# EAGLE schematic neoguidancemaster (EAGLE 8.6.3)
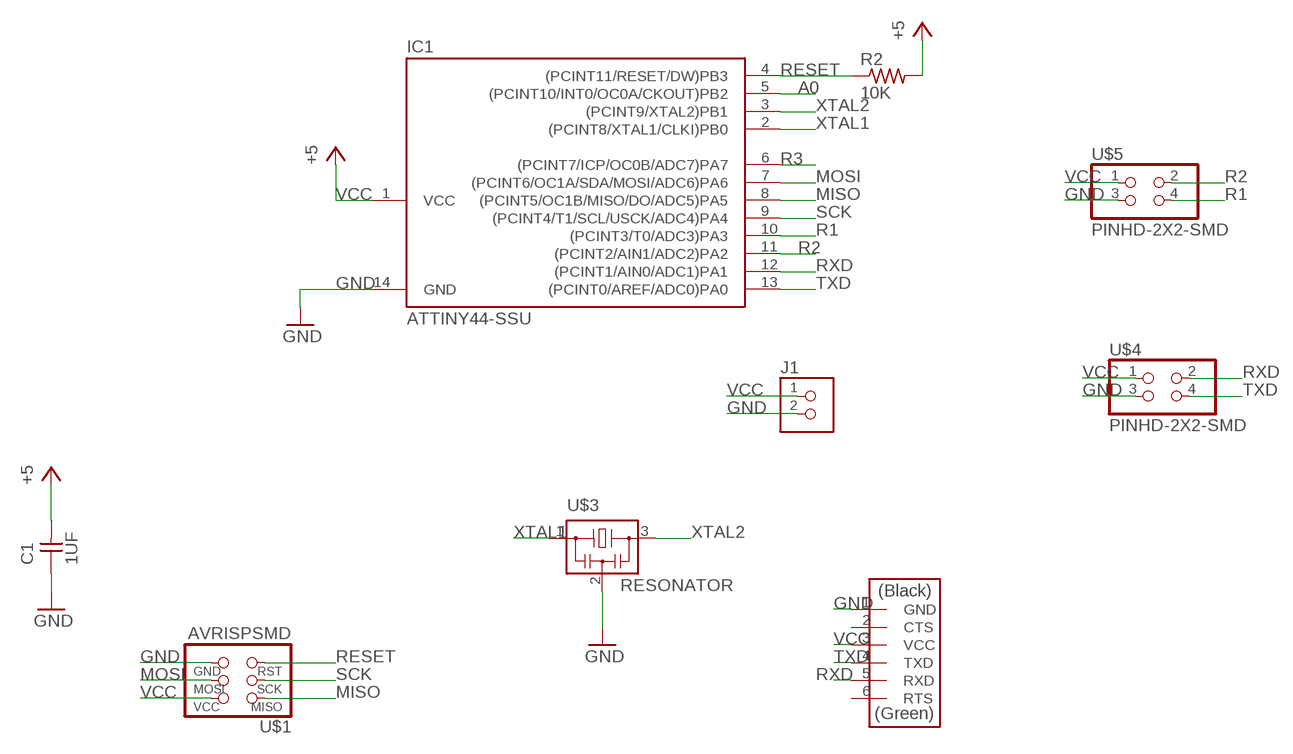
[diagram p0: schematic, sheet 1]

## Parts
C1  1UF  CAP-UNPOLARIZEDFAB  [C1206FAB]
IC1  ATTINY44-SSU  [SOIC14]
J1  TERM-1X02-ADAFRUIT  [3.5MMTERM]
R2  10K  RES-US1206FAB  [R1206FAB]
U$1  AVRISPSMD  [2X03SMD]
U$2  FTDI-SMD-HEADER  [1X06SMD]
U$3  RESONATOR  [EFOBM]
U$4  PINHD-2X2-SMD  [2X02SMD]
U$5  PINHD-2X2-SMD  [2X02SMD]

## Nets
A0: IC1.5((PCINT10/INT0/OC0A/CKOUT)PB2)
GND: C1.1 IC1.14(GND) J1.2 U$1.6(GND) U$2.1(GND) U$3.2 U$4.3 U$5.3
MISO: IC1.8((PCINT5/OC1B/MISO/DO/ADC5)PA5) U$1.1(MISO)
MOSI: IC1.7((PCINT6/OC1A/SDA/MOSI/ADC6)PA6) U$1.4(MOSI)
R1: IC1.10((PCINT3/T0/ADC3)PA3) U$5.4
R2: IC1.11((PCINT2/AIN1/ADC2)PA2) U$5.2
R3: IC1.6((PCINT7/ICP/OC0B/ADC7)PA7)
RESET: IC1.4((PCINT11/RESET/DW)PB3) R2.1 U$1.5(RST)
RXD: IC1.12((PCINT1/AIN0/ADC1)PA1) U$2.5(RXD) U$4.2
SCK: IC1.9((PCINT4/T1/SCL/USCK/ADC4)PA4) U$1.3(SCK)
TXD: IC1.13((PCINT0/AREF/ADC0)PA0) U$2.4(TXD) U$4.4
VCC: C1.2 IC1.1(VCC) J1.1 R2.2 U$1.2(VCC) U$2.3(VCC) U$4.1 U$5.1 ; supply symbol labelled +5
XTAL1: IC1.2((PCINT8/XTAL1/CLKI)PB0) U$3.1
XTAL2: IC1.3((PCINT9/XTAL2)PB1) U$3.3
Unconnected: U$2.2(CTS) U$2.6(RTS)

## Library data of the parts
C1 = fab:CAP-UNPOLARIZED
IC1 = fab:ATTINY44
J1 = fab:TERM-1X02: 3.5mm terminal block, 2 positions ED555-2DS as found in the fablab inventory.
R2 = fab:RES-US: Resistor (US Symbol)
U$1 = fab:AVRISP
U$2 = fab:FTDI-SMD-HEADER
U$3 = fab:RESONATOR
U$4 U$5 = fab:PINHD-2X2-SMD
